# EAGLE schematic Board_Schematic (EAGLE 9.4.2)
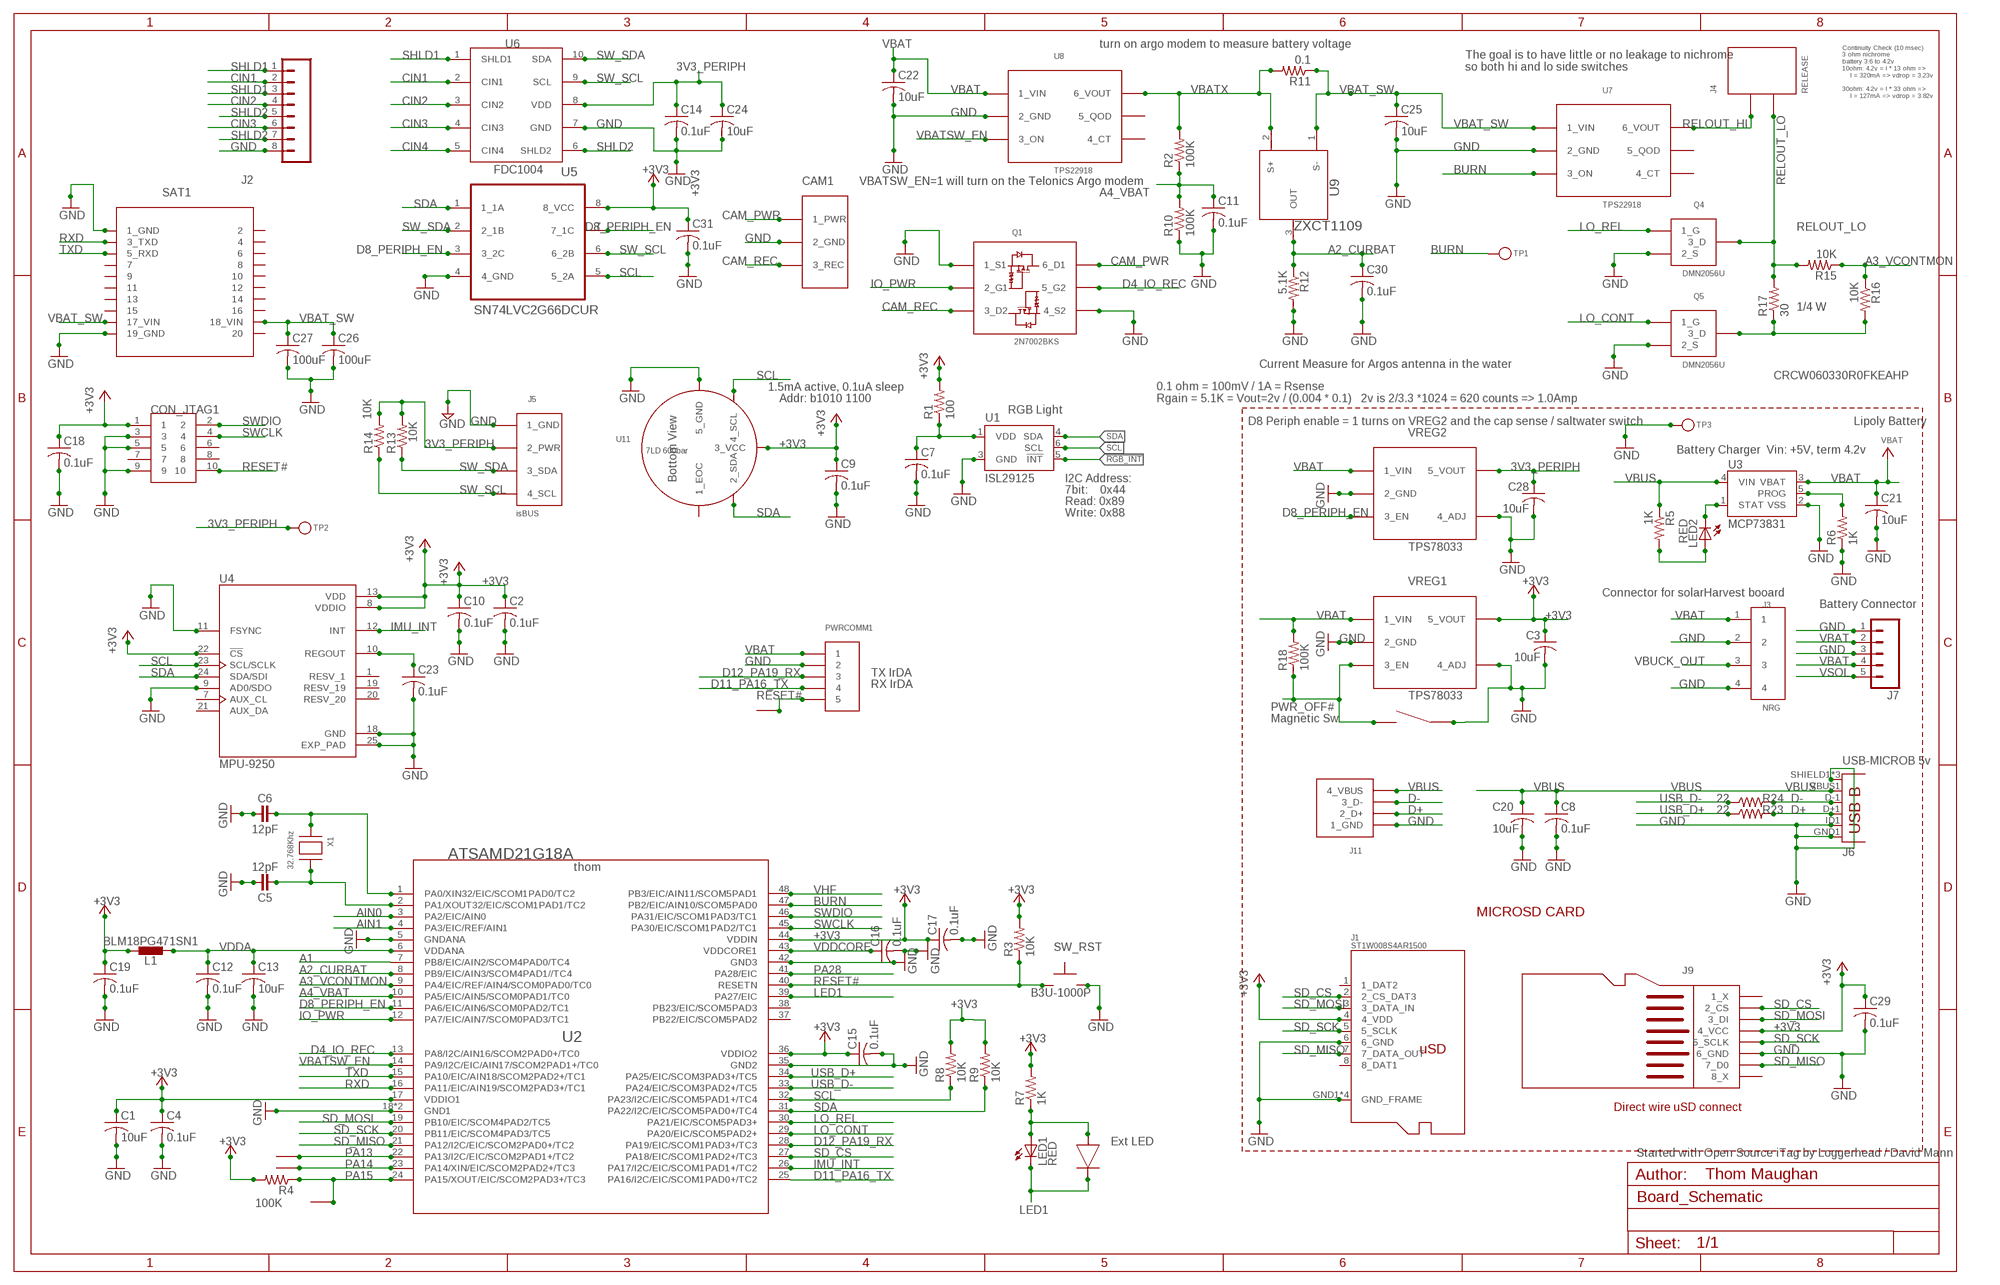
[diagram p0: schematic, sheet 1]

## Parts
C1  10uF  C-USC0603  [C0603]
C2  0.1uF  C-USC0402  [C0402]
C3  10uF  C-USC0603K  [C0603K]
C4  0.1uF  C-USC0402  [C0402]
C5  12pF  CAPACITORS-0402  [C0402]
C6  12pF  CAPACITORS-0402  [C0402]
C7  0.1uF  C-USC0402  [C0402]
C8  0.1uF  C-USC0402  [C0402]
C9  0.1uF  C-USC0402  [C0402]
C10  0.1uF  C-USC0402  [C0402]
C11  0.1uF  C-USC0402  [C0402]
C12  0.1uF  C-USC0402  [C0402]
C13  10uF  C-USC0603  [C0603]
C14  0.1uF  C-USC0402  [C0402]
C15  0.1uF  C-USC0402  [C0402]
C16  0.1uF  C-USC0402  [C0402]
C17  0.1uF  C-USC0402  [C0402]
C18  0.1uF  C-USC0402  [C0402]
C19  0.1uF  C-USC0402  [C0402]
C20  10uF  C-USC0603  [C0603]
C21  10uF  C-USC0603  [C0603]
C22  10uF  C-USC0603  [C0603]
C23  0.1uF  C-USC0402  [C0402]
C24  10uF  C-USC0603  [C0603]
C25  10uF  C-USC0603  [C0603]
C26  100uF  C-USC1210  [C1210]
C27  100uF  C-USC1210  [C1210]
C28  10uF  C-USC0603K  [C0603K]
C29  0.1uF  C-USC0402  [C0402]
C30  0.1uF  C-USC0402  [C0402]
C31  0.1uF  C-USC0402  [C0402]
CAM1  CON_1X3_CAMCTRL  [CON_1X3_CAMCTRL]
CON_JTAG1  HDR-SMT-50MIL/5X2  [HDR-SMT-50MIL/5X2]
J1  ST1W008S4AR1500  MICROSD_JAE_ST1W008S4AR1500  [MICROSD_JAE_ST1W008S4AR1500]
J2  CONN_08"  [1X08]
J3  NRG  CONNECTOR_1X4  [CONNECTOR_1X4_0_1]
J4  RELEASE  CON_1X2_0_1  [CON_1X2_0_1]
J5  isBUS  CON_ISBUS_0_1  [CON_1X4_0_1]
J6  USB-MICROB 5v  USB-MICROB"  [USB-B-MICRO-SMD_V03]
J7  M05PTH  [1X05]
J9  CON_8_MICROSD_WIRE  [CON_8_MICROSD_WIRE]
J11  CON_1X4_2MM_THRU  [CON_1X4_2MM_THRU]
L1  BLM18PG471SN1  INDUCTOR-0603  [C0603]
LED1  RED  LEDCHIPLED_0603  [CHIPLED_0603]
LED2  RED  LEDCHIPLED_0603  [CHIPLED_0603]
PWRCOMM1  CON_1X5_0_1  [CONNECTOR_1X5_0_1]
Q1  2N7002BKS  FET_N_DUAL_2N7002BKS  [SOT363]
Q4  DMN2056U  FET_A03414  [SOT23-3]
Q5  DMN2056U  FET_A03414  [SOT23-3]
R1  100  R-US_R0402  [R0402]
R2  100K  R-US_R0402  [R0402]
R3  10K  R-US_R0402  [R0402]
R4  100K  R-US_R0402  [R0402]
R5  1K  R-US_R0402  [R0402]
R6  1K  R-US_R0402  [R0402]
R7  1K  R-US_R0402  [R0402]
R8  10K  R-US_R0402  [R0402]
R9  10K  R-US_R0402  [R0402]
R10  100K  R-US_R0402  [R0402]
R11  0.1  R-US_R0603  [R0603]
R12  5.1K  R-US_R0402  [R0402]
R13  10K  R-US_R0402  [R0402]
R14  10K  R-US_R0402  [R0402]
R15  10K  R-US_R0402  [R0402]
R16  10K  R-US_R0402  [R0402]
R17  30  R-US_R0603  [R0603]
R18  100K  R-US_R0402  [R0402]
R23  22  R-US_R0402  [R0402]
R24  22  R-US_R0402  [R0402]
SAT1  TELONICS-ST-21H2-200A  [TELONICS_ST_21H2-200A]
SW_RST  B3U-1000P  [B3U-1000P]
TP1  TESTPOINTROUND1.5MM  [TESTPOINT_ROUND_1.5MM]
TP2  TESTPOINTROUND1.5MM  [TESTPOINT_ROUND_1.5MM]
TP3  TESTPOINTROUND1.5MM  [TESTPOINT_ROUND_1.5MM]
TP4  CON_1  [CON_1]
TP5  CON_1  [CON_1]
TP6  CON_1  [CON_1]
U1  ISL29125  [ODFN-LD-6]
U2  ATSAMD21G18A  [TQFN48_7MM]
U3  MCP73831  [SOT23-5]
U4  MPU-9250  MPU-9250-SNAP  [MPU-9250-FOOTPRINT]
U5  SN74LVC2G66DCUR  ANALOG_SW_SN74LVCG66DCUR  [ANALOG_SW_SN74LVCG66DCUR]
U6  FDC1004  [VSSOP-10]
U7  TPS22918  [SOT23-6]
U8  TPS22918  [SOT23-6]
U9  ZXCT1109  [SOT23]
U11  7LD 600bar  KELLER_7LD_PRESSURE  [KELLER_7LD]
U$3  CON_2_MAGSW  [CON_2_MAGSW]
U$4  CON_2_LED  [CON_2_LED]
U$5  CON_1  [CON_1]
VREG1  TPS78033  REG101  [SOT23-5]
VREG2  TPS78033  REG101  [SOT23-5]
X1  32.768Khz  XTAL_ABS06_32K  [XTAL_ABS06]

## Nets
3V3_PERIPH: C14.1 C24.1 C28.1 J5.P$2(2_PWR) R13.2 R14.2 TP2.P$1 U6.8(VDD) VREG2.P$5(5_VOUT)
!RGB_INT: U1.5(!INT)
+3V3: C1.1 C2.1 C3.1 C4.1 C9.1 C10.1 C15.1 C17.1 C18.1 C19.1 C29.1 C31.1 CON_JTAG1.1 J1.4(4_VDD) J9.4_VCC J9.P4(4_VCC) L1.2 R1.2 R3.2 R4.2 R7.2 R8.2 R9.2 U2.17(VDDIO1) U2.36(VDDIO2) U2.44(VDDIN) U4.8(VDDIO) U4.13(VDD) U4.22(!CS) U5.8(8_VCC) U11.3_VCC VREG1.P$5(5_VOUT)
A1: U2.7(PB8/EIC/AIN2/SCOM4PAD0/TC4)
A2_CURBAT: C30.1 R12.1 U2.8(PB9/EIC/AIN3/SCOM4PAD1//TC4) U9.3(OUT)
A3_VCONTMON: R15.1 R16.1 U2.9(PA4/EIC/REF/AIN4/SCOM0PAD0/TC0)
A4_VBAT: C11.1 R2.1 R10.2 U2.10(PA5/EIC/AIN5/SCOM0PAD1/TC0)
AIN0: U2.3(PA2/EIC/AIN0)
AIN1: U2.4(PA3/EIC/REF/AIN1)
BURN: TP1.P$1 U2.47(PB2/EIC/AIN10/SCOM5PAD0) U7.3(3_ON)
CAM_PWR: CAM1.1_PWR Q1.6(6_D1)
CAM_REC: CAM1.3_REC Q1.3(3_D2)
CIN1: J2.2 U6.2(CIN1)
CIN2: J2.4 U6.3(CIN2)
CIN3: J2.6 U6.4(CIN3)
CIN4: U6.5(CIN4)
D4_IO_REC: Q1.5(5_G2) U2.13(PA8/I2C/AIN16/SCOM2PAD0+/TC0)
D8_PERIPH_EN: U2.11(PA6/EIC/AIN6/SCOM0PAD2/TC1) U5.3(3_2C) U5.7(7_1C) VREG2.P$3(3_EN)
D11_PA16_TX: PWRCOMM1.4 U2.25(PA16/I2C/EIC/SCOM1PAD0+/TC2)
D12_PA19_RX: PWRCOMM1.3 U2.28(PA19/EIC/SCOM1PAD3+/TC3)
D+ [USBpair]: J6.D+1(D+) J11.P$2(2_D+) R23.2
D- [USBpair]: J6.D-1(D-) J11.P$3(3_D-) R24.2
GND [gnd]: C1.2 C2.2 C3.2 C4.2 C5.2 C6.1 C7.2 C8.2 C9.2 C10.2 C11.2 C12.2 C13.2 C14.2 C15.2 C16.2 C17.2 C18.2 C19.2 C20.2 C21.2 C22.2 C23.2 C24.2 C25.2 C26.2 C27.2 C28.2 C29.2 C30.2 C31.2 CAM1.2_GND CON_JTAG1.3 CON_JTAG1.5 CON_JTAG1.9 J1.6(6_GND) J1.GND1(GND_FRAME) J1.GND2(GND_FRAME) J1.GND3(GND_FRAME) J1.GND4(GND_FRAME) J2.8 J3.2 J3.4 J5.P$1(1_GND) J6.GND1(GND) J6.ID1(USBID) J6.SHIELD1(SHIELD) J6.SHIELD2(SHIELD) J6.SHIELD3(SHIELD) J7.1 J7.3 J9.6_GND J9.P6(6_GND) J11.P$1(1_GND) PWRCOMM1.2 Q1.1(1_S1) Q1.4(4_S2) Q4.2(2_S) Q5.2(2_S) R6.1 R10.1 R12.2 SAT1.1(1_GND) SAT1.19(19_GND) SAT1.21(1_GND) SAT1.39(19_GND) SW_RST.P$2 TP3.P$1 U1.3(GND) U2.5(GNDANA) U2.18(GND1) U2.35(GND2) U2.42(GND3) U2.THERMAL(GND1) U3.2(VSS) U4.9(AD0/SDO) U4.11(FSYNC) U4.18(GND) U4.25(EXP_PAD) U5.4(4_GND) U6.7(GND) U7.2(2_GND) U8.2(2_GND) U11.5_GND U$3.2 VREG1.P$2(2_GND) VREG1.P$4(4_ADJ) VREG2.P$2(2_GND) VREG2.P$4(4_ADJ)
IMU_INT: U2.26(PA17/I2C/EIC/SCOM1PAD1+/TC2) U4.12(INT)
IO_PWR: Q1.2(2_G1) U2.12(PA7/EIC/AIN7/SCOM0PAD3/TC1)
LAN: LED1.A R7.1 U$4.P$1(1A)
LED1: LED1.C U2.39(PA27/EIC) U$4.P$2(2K)
LO_CONT: Q5.1(1_G) U2.29(PA20/EIC/SCOM5PAD2+)
LO_REL: Q4.1(1_G) U2.30(PA21/EIC/SCOM5PAD3+)
N$1: C6.2 U2.1(PA0/XIN32/EIC/SCOM1PAD0/TC2) X1.P$1
N$2: LED2.C U3.1(STAT)
N$3: LED2.A R5.2
N$4: R6.2 U3.5(PROG)
N$7: C7.1 R1.1 U1.1(VDD)
N$8: C5.1 U2.2(PA1/XOUT32/EIC/SCOM1PAD1/TC2) X1.P$2
N$11: Q5.3(3_D) R16.2 R17.1
N$16: C23.1 U4.10(REGOUT)
PA13: TP4.P$1 U2.22(PA13/I2C/EIC/SCOM2PAD1+/TC2)
PA14: TP5.P$1 U2.23(PA14/XIN/EIC/SCOM2PAD2+/TC3)
PA15: R4.1 TP6.P$1 U2.24(PA15/XOUT/EIC/SCOM2PAD3+/TC3)
PA28: U2.41(PA28/EIC)
PWR_OFF#: R18.1 U$3.1 VREG1.P$3(3_EN)
RELOUT_HI: J4.P$1 U7.6(6_VOUT)
RELOUT_LO: J4.P$2 Q4.3(3_D) R15.2 R17.2
RESET#: CON_JTAG1.10 PWRCOMM1.5 R3.1 SW_RST.P$1 U2.40(RESETN) U$5.P$1
RXD: SAT1.3(3_TXD) SAT1.23(3_TXD) U2.16(PA11/EIC/AIN19/SCOM2PAD3+/TC1)
SCL: R8.1 U1.6(SCL) U2.32(PA23/I2C/EIC/SCOM5PAD1+/TC4) U4.23(SCL/SCLK) U5.5(5_2A) U11.4_SCL
SD_CS: J1.2(2_CS_DAT3) J9.2_CS J9.P2(2_CS) U2.27(PA18/EIC/SCOM1PAD2+/TC3)
SD_MISO: J1.7(7_DATA_OUT) J9.7_DO(7_D0) J9.P7(7_D0) U2.21(PA12/I2C/EIC/SCOM2PAD0+/TC2)
SD_MOSI: J1.3(3_DATA_IN) J9.3_DI J9.P3(3_DI) U2.19(PB10/EIC/SCOM4PAD2/TC5)
SD_SCK: J1.5(5_SCLK) J9.5_SCK(5_SCLK) J9.P5(5_SCLK) U2.20(PB11/EIC/SCOM4PAD3/TC5)
SDA: R9.1 U1.4(SDA) U2.31(PA22/I2C/EIC/SCOM5PAD0+/TC4) U4.24(SDA/SDI) U5.1(1_1A) U11.2_SDA
SHLD1: J2.1 J2.3 U6.1(SHLD1)
SHLD2: J2.5 J2.7 U6.6(SHLD2)
SW_SCL: J5.P$4(4_SCL) R14.1 U5.6(6_2B) U6.9(SCL)
SW_SDA: J5.P$3(3_SDA) R13.1 U5.2(2_1B) U6.10(SDA)
SWCLK: CON_JTAG1.4 U2.45(PA30/EIC/SCOM1PAD2/TC1)
SWDIO: CON_JTAG1.2 U2.46(PA31/EIC/SCOM1PAD3/TC1)
TXD: SAT1.5(5_RXD) SAT1.25(5_RXD) U2.15(PA10/EIC/AIN18/SCOM2PAD2+/TC1)
USB_D+ [USBpair]: R23.1 U2.34(PA25/EIC/SCOM3PAD3+/TC5)
USB_D- [USBpair]: R24.1 U2.33(PA24/EIC/SCOM3PAD2+/TC5)
VBAT: C21.1 C22.1 J3.1 J7.2 J7.4 PWRCOMM1.1 R18.2 U3.3(VBAT) U8.1(1_VIN) VREG1.P$1(1_VIN) VREG2.P$1(1_VIN)
VBAT_SW: C25.1 C26.1 C27.1 R11.1 SAT1.17(17_VIN) SAT1.18(18_VIN) SAT1.37(17_VIN) SAT1.38(18_VIN) U7.1(1_VIN) U9.1(S-)
VBATSW_EN: U2.14(PA9/I2C/EIC/AIN17/SCOM2PAD1+/TC0) U8.3(3_ON)
VBATX: R2.2 R11.2 U8.6(6_VOUT) U9.2(S+)
VBUCK_OUT: J3.3
VBUS: C8.1 C20.1 J6.VBUS1(VBUS) J11.P$4(4_VBUS) R5.1 U3.4(VIN)
VDDA: C12.1 C13.1 L1.1 U2.6(VDDANA)
VDDCORE: C16.1 U2.43(VDDCORE1)
VHF: U2.48(PB3/EIC/AIN11/SCOM5PAD1)
VSOL: J7.5
Unconnected: CON_JTAG1.6 CON_JTAG1.7 CON_JTAG1.8 J1.1(1_DAT2) J1.8(8_DAT1) J9.1_X J9.8_X J9.P1(1_X) J9.P8(8_X) SAT1.2 SAT1.4 SAT1.6 SAT1.7 SAT1.8 SAT1.9 SAT1.10 SAT1.11 SAT1.12 SAT1.13 SAT1.14 SAT1.15 SAT1.16 SAT1.20 SAT1.22 SAT1.24 SAT1.26 SAT1.27 SAT1.28 SAT1.29 SAT1.30 SAT1.31 SAT1.32 SAT1.33 SAT1.34 SAT1.35 SAT1.36 SAT1.40 U2.37(PB22/EIC/SCOM5PAD2) U2.38(PB23/EIC/SCOM5PAD3) U4.1(RESV_1) U4.7(AUX_CL) U4.19(RESV_19) U4.20(RESV_20) U4.21(AUX_DA) U7.4(4_CT) U7.5(5_QOD) U8.4(4_CT) U8.5(5_QOD) U11.1_EOC

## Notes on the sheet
- turn on argo modem to measure battery voltage
- The goal is to have little or no leakage to nichrome
  so both hi and lo side switches
- Continuity Check (10 msec)
  3 ohm nichrome
  battery 3.6 to 4.2v
  10ohm: 4.2v = I * 13 ohm =>
      I = 320mA => vdrop = 3.23v 
  
  30ohm: 4.2v = I * 33 ohm =>
      I = 127mA => vdrop = 3.82v
- VBATSW_EN=1 will turn on the Telonics Argo modem
- 1/4 W
- Current Measure for Argos antenna in the water
- CRCW060330R0FKEAHP
- 1.5mA active, 0.1uA sleep
- Addr: b1010 1100
- 0.1 ohm = 100mV / 1A = Rsense
  Rgain = 5.1K = Vout=2v / (0.004 * 0.1)   2v is 2/3.3 *1024 = 620 counts => 1.0Amp
- RGB Light
- D8 Periph enable = 1 turns on VREG2 and the cap sense / saltwater switch | Lipoly Battery
- Battery Charger  Vin: +5V, term 4.2v
- I2C Address:
- 7bit:    0x44
- Read: 0x89
- Write: 0x88
- Connector for solarHarvest booard
- Battery Connector
- TX IrDA
- RX IrDA
- Magnetic Sw
- MICROSD CARD
- Direct wire uSD connect
- Ext LED
- Started with Open Source iTag by Loggerhead / David Mann
- Thom Maughan

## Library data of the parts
C1 C2 C4 C7-C25 C29-C31 = iss_whalesharktag_v1_1:C-US: CAPACITOR, American symbol
C3 C26-C28 = iss_subg2cell_v3_0:C-US: CAPACITOR, American symbol
C5 C6 = iss_whalesharktag_v1_1:CAPACITORS: Capacitors
CAM1 = thomz:CON_1X3_CAMCTRL
CON_JTAG1 = iss_whalesharktag_v1_1:HDR-SMT-50MIL/5X2
J1 = iss_whalesharktag_v1_1:MICROSD_JAE_ST1W008S4AR1500: JAE ST1W008S4AR1500
J2 = SparkFun-Connectors:CONN_08: Multi connection point. Often used as Generic Header-pin footprint for 0.1 inch spaced/style header connections On any of the 0.1 inch spaced packages, you can populate with these: Break Away Headers - Straight (PRT-00116) Break Away Male Headers - Right Angle (PRT-00553) Female Headers (PRT-00115)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; PROD_ID: CONN-08438
J3 = thomz:CONNECTOR_1X4
J4 = thomz:CON_1X2_0_1
J5 = iss_subg2cell_v3_0:CON_ISBUS_0_1
J6 = iss_subg2cell_v3_0:USB-MICROB; PROD_ID: CONN-11752
J7 = iss_whalesharktag_v1_1:M05: Header 5 Standard 5-pin 0.1" header. Use with straight break away headers (SKU : PRT-00116), right angle break away headers (PRT-00553), swiss pins (PRT-00743), machine pins (PRT-00117), and female headers (PRT-00115). Molex polarized connector foot print use with SKU : PRT-08230 with associated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
J9 = iss_whalesharktag_v1_1:CON_8_MICROSD_WIRE
J11 = iss_whalesharktag_v1_1:CON_1X4_2MM_THRU
L1 = iss_whalesharktag_v1_1:INDUCTOR: Inductors
LED1 LED2 = iss_whalesharktag_v1_1:LED: LED
PWRCOMM1 = thomz:CON_1X5_0_1
Q1 = thomz:FET_N_DUAL_2N7002BKS
Q4 Q5 = thomz:FET_A03414
R1-R10 R12-R16 R18 R23 R24 = iss_whalesharktag_v1_1:R-US_: RESISTOR, American symbol
R11 R17 = resistor:R-US_: RESISTOR, American symbol
SAT1 = iss_whalesharktag_v1_1:TELONICS-ST-21H2-200A
SW_RST = iss_whalesharktag_v1_1:B3U-1000P
TP1-TP3 = iss_whalesharktag_v1_1:TESTPOINT: Test Point
TP4-TP6 U$5 = thomz:CON_1
U1 = iss_whalesharktag_v1_1:ISL29125: The ISL29125 is a low power, high sensitivity RGB color light sensor with an I2C interface.
U2 = iss_whalesharktag_v1_1:ATSAMD21G18A
U3 = iss_whalesharktag_v1_1:MCP73831: Microchip's MCP73831 Miniature single cell, fully integrated Li-Ion, Li-polymer charge management controller http://ww1.microchip.com/downloads/en/DeviceDoc/21984a.pdf
U4 = iss_whalesharktag_v1_1:MPU-9250-SNAP
U5 = thomz:ANALOG_SW_SN74LVCG66DCUR
U6 = circuitects:FDC1004
U7 U8 = iss_whalesharktag_v1_1:TPS22918
U9 = thomz:ZXCT1109
U11 = iss_whalesharktag_v1_1:KELLER_7LD_PRESSURE
U$3 = thomz:CON_2_MAGSW
U$4 = thomz:CON_2_LED
VREG1 VREG2 = iss_subg2cell_v3_0:REG101
X1 = iss_whalesharktag_v1_1:XTAL_ABS06_32K

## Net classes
1 USB: width 0.102 mm, drill 0.1 mm
2 gnd: width 0.102 mm, drill 0.1 mm
3 usbvcc: width 0.102 mm, drill 0.1 mm, clearance 0.15 mm
4 USBpair: width 0.102 mm, drill 0.1 mm, clearance 0.15 mm to class 3

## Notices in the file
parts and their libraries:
SparkFun-Connectors: Licensing: Creative Commons ShareAlike 4.0 International - https://creativecommons.org/licenses/by-sa/4.0
